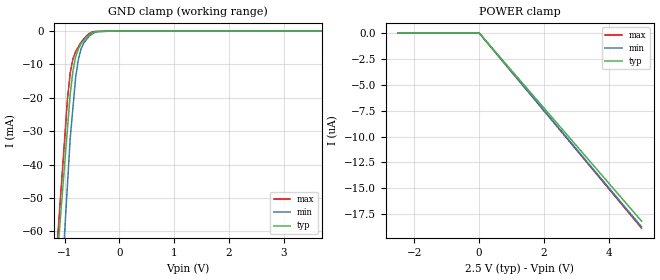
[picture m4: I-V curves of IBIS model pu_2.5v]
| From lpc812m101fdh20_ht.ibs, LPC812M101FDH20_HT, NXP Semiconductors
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[Model] pu_2.5v
Model_type Input
Vinl = 750.000mV
Vinh = 1.75000V
C_comp 909.000fF 904.000fF 914.000fF
| variable typ   min   max
[Voltage Range] 2.50000V 2.25000V 2.75000V
[POWER Clamp Reference] 2.50000V 2.25000V 2.75000V
[GND Clamp Reference] 0.00000V 0.00000V 0.00000V
[Temperature Range]   25   105   -40
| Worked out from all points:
|   GND clamp passes 1 mA (typ) near -0.54 V on its own axis
[GND Clamp]
-2.5V     -349.8mA   -474.9mA   -378.6mA
-950mV    -29.07mA   -45.83mA   -20.26mA
-900mV    -18.72mA   -31.99mA   -12.43mA
-850mV    -11.92mA   -22.84mA   -8.272mA
-800mV    -7.671mA   -13.7mA    -6.085mA
-750mV    -5.233mA   -8.393mA   -4.695mA
-700mV    -3.729mA   -5.238mA   -3.305mA
-650mV    -2.754mA   -3.531mA   -2.353mA
-500mV    -508.2uA   -915.1uA   -281.2uA
-400mV    -162.5uA   -153.2uA   -88.55uA
-200mV    -39.32uA   -30.88uA   -47.58uA
5V        0A         0A         0A
[POWER Clamp]
-2.5V     0A         0A         0A
0V        0A         0A         0A
5V        -18.17uA   -18.71uA   -18.84uA
